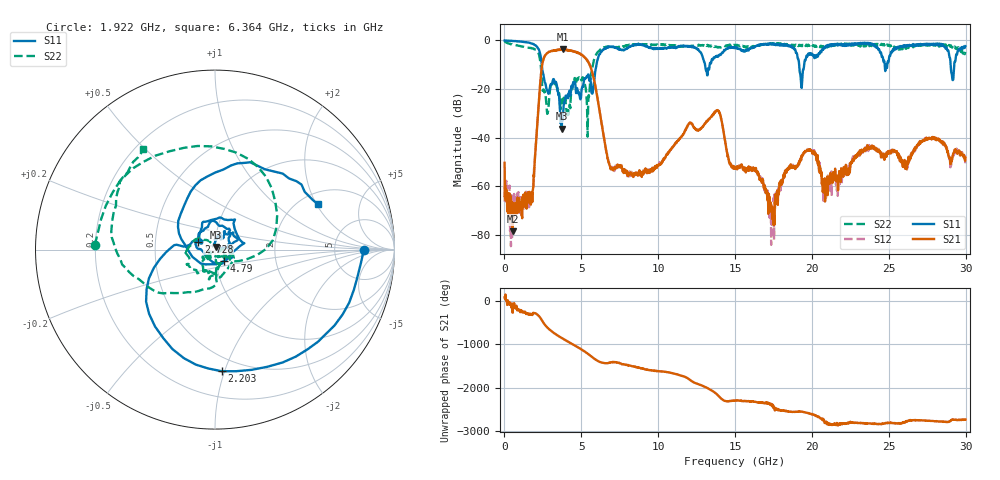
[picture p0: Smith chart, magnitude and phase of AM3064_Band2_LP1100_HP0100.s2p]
# Hz S DB R 50.0
!freq dBS11 angS11 dBS21 angS21 dBS12 angS12 dBS22 angS22
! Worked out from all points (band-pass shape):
!   1600 points, 10 MHz to 29.98 GHz, reference 50 ohm
!   highest |S21| = -3.71 dB at 3.777 GHz (marker M1); lowest = -78.5 dB at 534.8 MHz (marker M2)
!   |S21| within 3 dB of the highest: 2.597 GHz to 5.185 GHz (2.588 GHz wide, 66.5 % of centre)
!   lowest |S11| = -36.3 dB at 3.721 GHz (marker M3), VSWR 1.03, Z = 50.5 + j1.44 ohm
!   |S11| at or under -10 dB: 2.426 GHz to 5.984 GHz (3.558 GHz wide, 84.6 % of centre); 13.05 GHz to 13.35 GHz (304.1 MHz wide, 2.3 % of centre); 19.17 GHz to 19.49 GHz (324.1 MHz wide, 1.68 % of centre)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
!   |S22| runs from -39.6 to -0.3 dB; largest |S21 - S12| = 0.014
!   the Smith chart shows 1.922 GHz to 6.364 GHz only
!   S11 on the Smith chart (normalised r, x): 1.922 GHz: 11, +0; 2.203 GHz: 0.39, -0.98; 2.728 GHz: 0.83, +0.07; 4.79 GHz: 1.10, -0.14; 6.364 GHz: 2.48, +2.06
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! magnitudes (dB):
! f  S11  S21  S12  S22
! 10 MHz  0.0  -50.3  -66.2  -0.3
! 534.8 MHz  -0.2  -78.5  -76.3  -1.6
! 1.922 GHz  -1.6  -56.1  -52.7  -3.5
! 2.203 GHz  -3.4  -27.9  -27.9  -5.1
! 2.728 GHz  -19.7  -5.6  -5.5  -26.2
! 3.721 GHz  -36.3  -3.8  -3.7  -24.3
! 3.777 GHz  -32.9  -3.7  -3.8  -26.7
! 4.79 GHz  -21.7  -5.0  -5.0  -15.8
! 5.015 GHz  -20.3  -5.9  -5.8  -16.4
! 5.408 GHz  -14.4  -8.3  -8.4  -39.6
! 6.364 GHz  -4.1  -35.8  -35.7  -3.2
! 6.983 GHz  -2.6  -52.8  -51.9  -2.7
! 10 GHz  -3.4  -51.4  -51.1  -1.8
! 13.82 GHz  -6.3  -28.7  -28.7  -2.7
! 15 GHz  -2.9  -52.7  -52.6  -1.9
! 16.43 GHz  -2.1  -53.8  -54.5  -2.1
! 17.39 GHz  -1.5  -68.1  -75.7  -1.3
! 19.33 GHz  -19.5  -47.9  -47.3  -2.1
! 19.99 GHz  -5.5  -45.3  -45.3  -1.8
! 20.82 GHz  -2.8  -62.6  -57.4  -2.3
! 25 GHz  -8.2  -46.6  -45.8  -1.8
! 29.98 GHz  -2.4  -48.2  -50.5  -4.7
